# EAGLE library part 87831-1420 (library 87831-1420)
Header 2.00mm Milli-Grid, vert, TH, 14w Molex MILLI-GRID Series, Series Number 87831, 2mm Pitch 14 Way 2 Row Straight PCB Header, Solder Termination, 2A Source: Datasheet
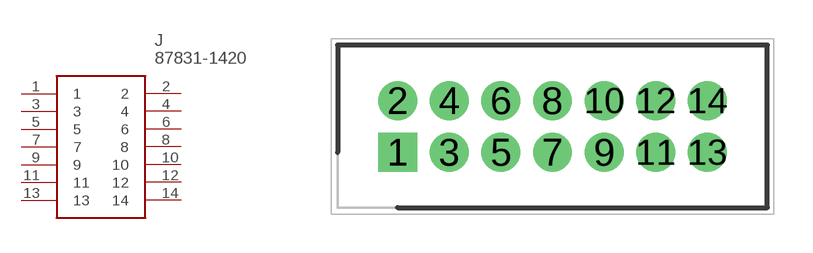
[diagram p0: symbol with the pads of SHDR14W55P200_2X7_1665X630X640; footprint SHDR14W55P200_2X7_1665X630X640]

Designator prefix J

## 87831-1420 (Description: Header 2.00mm Milli-Grid, vert, TH, 14w Molex MILLI-GRID Series, Series Number 87831, 2mm Pitch 14 Way 2 Row Straight PCB Header, Solder Termination, 2A; Height: 6.4mm; Manufacturer_Name: Molex; Manufacturer_Part_Number: 87831-1420; Mouser_Part_Number: 538-87831-1420; Mouser_Price-Stock: https://www.mouser.co.uk/ProductDetail/Molex/87831-1420?qs=QtQX4uD3c2VDCL534TqpVg%3D%3D)  [SHDR14W55P200_2X7_1665X630X640]
1  1
2  2
3  3
4  4
5  5
6  6
7  7
8  8
9  9
10  10
11  11
12  12
13  13
14  14

## Footprint SHDR14W55P200_2X7_1665X630X640 (pad centres in mm)
87831-1420
drill 1 pad 1.5 square: 1 0,0
drill 1 pad 1.5: 2 0,2; 3 2,0; 4 2,2; 5 4,0; 6 4,2; 7 6,0; 8 6,2; 9 8,0; 10 8,2; 11 10,0; 12 10,2; 13 12,0; 14 12,2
